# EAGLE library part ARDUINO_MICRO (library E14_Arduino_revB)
Device for representing an Arduino Micro board with a footprint in an EAGLE design. Created by Dave Young for Element14. More EAGLE documentation at: http://www.element14.com/community/community/knode/cadsoft_eagle
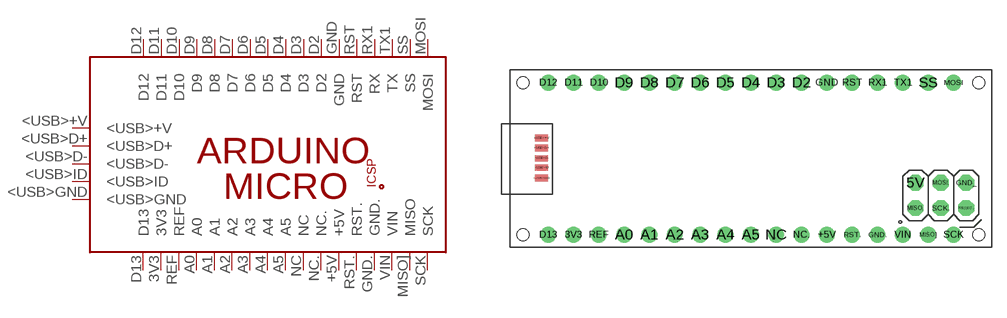
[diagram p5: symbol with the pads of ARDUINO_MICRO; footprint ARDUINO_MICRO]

Designator prefix PCB

## ARDUINO_MICRO  [ARDUINO_MICRO]
3V3  3V3
5V  5V
+5V  +5V
<USB>+V  <USB>+V
<USB>D+  <USB>D+
<USB>D-  <USB>D-
<USB>GND  <USB>GND
<USB>ID  <USB>ID
A0  A0
A1  A1
A2  A2
A3  A3
A4  A4
A5  A5
D2  D2
D3  D3
D4  D4
D5  D5
D6  D6
D7  D7
D8  D8
D9  D9
D10  D10
D11  D11
D12  D12
D13  D13
GND  GND
GND.  GND.
GND_  GND_
MISO.  MISO.
MISO]  MISO
MOSI  MOSI
MOSI.  MOSI.
NC  NC
NC.  NC.
REF  REF
RESET..  RESET..
RST  RST
RST.  RST.
RX1  RX
SCK  SCK
SCK.  SCK.
SS  SS
TX1  TX
VIN  VIN

## Footprint ARDUINO_MICRO (pad centres in mm)
Footprint for representing an Arduino Micro board in an EAGLE schematic. Created by Dave Young for Element14. More EAGLE documentation at: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
drill 1.016 pad 1.575: 3V3 6.35,1.27; +5V 31.75,1.27; A0 11.43,1.27; A1 13.97,1.27; A2 16.51,1.27; A3 19.05,1.27; A4 21.59,1.27; A5 24.13,1.27; D2 29.21,16.51; D3 26.67,16.51; D4 24.13,16.51; D5 21.59,16.51; D6 19.05,16.51; D7 16.51,16.51; D8 13.97,16.51; D9 11.43,16.51; D10 8.89,16.51; D11 6.35,16.51; D12 3.81,16.51; D13 3.81,1.27; GND 31.75,16.51; GND. 36.83,1.27; MISO] 41.91,1.27; MOSI 44.45,16.51; NC 26.67,1.27; NC. 29.21,1.27; REF 8.89,1.27; RST 34.29,16.51; RST. 34.29,1.27; RX1 36.83,16.51; SCK 44.45,1.27; SS 41.91,16.51; TX1 39.37,16.51; VIN 39.37,1.27
drill 1.016 pad 1.575 octagon: 5V 40.64,6.477; GND_ 45.72,6.477; MISO. 40.64,3.937; MOSI. 43.18,6.477; RESET.. 45.72,3.937; SCK. 43.18,3.937
smd 1.27 x 0.635: <USB>+V 3.15,10.947; <USB>D+ 3.15,9.957; <USB>D- 3.15,8.941; <USB>GND 3.15,6.96; <USB>ID 3.15,7.976
hole 1.2 at 1.27,1.27
hole 1.2 at 1.27,16.51
hole 1.2 at 46.99,16.51
hole 1.2 at 46.99,1.27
